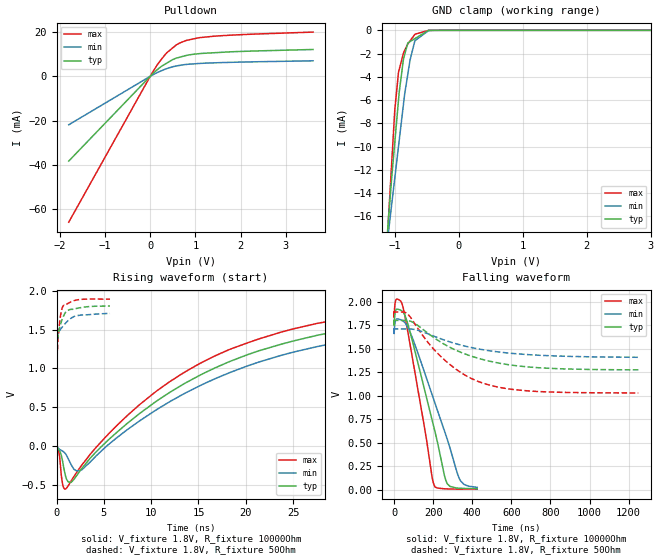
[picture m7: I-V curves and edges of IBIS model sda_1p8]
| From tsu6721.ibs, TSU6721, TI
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|   sda_1p8 Model
[Model]   sda_1p8
Model_type   I/O_open_drain
Polarity   Non-Inverting
Enable   Active-High
Vinl = 0.54
Vinh = 1.26
Vmeas = 0.9
Vref = 1.8
Cref = 35pF
Rref = 10000
|   typ   min   max
C_comp   1.376e-12   1.221e-12   1.514e-12
[Model spec]
|subparameter
Vinl   0.54   0.513   0.567
Vinh   1.26   1.197   1.323
[Voltage Range]   1.8   1.71   1.89
|Ambient Temperature   25   85   -40
|Junction Temperature
[Temperature Range]   27   125   -40
[Pullup Reference]   1.8   1.71   1.89
[Pulldown Reference]   0   0   0
[Power Clamp Reference]   1.8   1.71   1.89
[GND Clamp Reference]   0   0   0
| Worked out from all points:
|   slope of the pulldown table from 0 to 0.27 V, typ, clamps not added: 56.5 ohm
|   GND clamp passes 1 mA (typ) near -0.77 V on its own axis
|   falling waveform, V_fixture 1.8V, R_fixture 10000Ohm: 20-80 % time 125ns typ, 162ns min, 92.3ns max; typ from 1.8 V to 0.01 V
|   rising waveform, V_fixture 1.8V, R_fixture 10000Ohm: 20-80 % time 19.9ns typ, 21.8ns min, 17.8ns max; typ from 0.009 V to 1.8 V
|   falling waveform, V_fixture 1.8V, R_fixture 50Ohm: 20-80 % time 309ns typ, 337ns min, 257ns max; typ from 1.8 V to 1.27 V
|   rising waveform, V_fixture 1.8V, R_fixture 50Ohm: 20-80 % time 717ps typ, 1.33ns min, 398ps max; typ from 1.27 V to 1.8 V
[Pulldown]
|   Voltage   I(typ)   I(min)   I(max)
-1.8V     -38.2mA    -21.84mA   -65.75mA
35.91mV   716.9uA    418.8uA    1.294mA
168.2mV   3.206mA    1.819mA    5.583mA
332.6mV   5.544mA    3.231mA    9.865mA
574.6mV   8.199mA    4.667mA    14.12mA
797.6mV   9.416mA    5.363mA    16.19mA
1.058V    10.18mA    5.763mA    17.33mA
1.382V    10.6mA     6.059mA    18.03mA
3.6V      12.09mA    6.997mA    19.94mA
[GND Clamp]
|   Voltage   I(typ)   I(min)   I(max)
-1.8V     -71.23mA   -53.99mA   -101.6mA
-1.165V   -21.26mA   -20.52mA   -23.91mA
-1.096V   -16.21mA   -17.32mA   -16.16mA
-1.044V   -12.54mA   -14.88mA   -11.22mA
-999.8mV  -9.773mA   -12.81mA   -7.043mA
-939.3mV  -5.987mA   -9.974mA   -3.59mA
-862.2mV  -2.474mA   -6.361mA   -1.972mA
-793.8mV  -1.081mA   -3.757mA   -1.169mA
-759.2mV  -966.1uA   -2.551mA   -910.4uA
-682.3mV  -709.7uA   -893.4uA   -334.1uA
-434.3mV  -4.616uA   -12.32uA   -1.347uA
3.6V      0A         0A         0A
[POWER Clamp]
|   Voltage   I(typ)   I(min)   I(max)
-1.8V     0A         0A         0A
0V        0A         0A         0A
3.6V      0A         0A         0A
[Ramp]
R_load = 10000
|   typ   min   max
dV/dt_r   1.07486/1.99435e-08   1.01737/2.21728e-08   1.13092/1.78159e-08
dV/dt_f   1.07441/1.25188e-07   1.01502/1.6283e-07   1.13085/9.2297e-08
[Falling Waveform]
V_fixture = 1.8V
V_fixture_min = 1.71V
V_fixture_max = 1.89V
R_fixture = 10000Ohm
|   Time   V(typ)   V(min)   V(max)
0s        1.8V       1.71V      1.89V
200ps     1.747V     1.66V      1.832V
5.275ns   1.878V     1.777V     1.983V
13.03ns   1.92V      1.815V     2.027V
47.75ns   1.885V     1.792V     1.925V
96.45ns   1.561V     1.6V       1.371V
207.4ns   634.4mV    932mV      37.15mV
272.2ns   62.63mV    535.6mV    8.087mV
339.5ns   14.97mV    95.52mV    6.075mV
425.1ns   10.34mV    24.6mV     5.437mV
[Rising Waveform]
V_fixture = 1.8V
V_fixture_min = 1.71V
V_fixture_max = 1.89V
R_fixture = 10000Ohm
|   Time   V(typ)   V(min)   V(max)
0s        8.562mV    14.37mV    5.137mV
650ps     -195.2mV   -62.19mV   -491.8mV
925ps     -367.8mV   -92.12mV   -550mV
1.5ns     -464.7mV   -224.7mV   -453.8mV
2.625ns   -291.7mV   -303.7mV   -248.8mV
12ns      695.6mV    576mV      833.3mV
18.4ns    1.094V     951.8mV    1.25V
27.58ns   1.427V     1.282V     1.58V
45.83ns   1.705V     1.579V     1.83V
76.27ns   1.796V     1.698V     1.891V
[Falling Waveform]
V_fixture = 1.8V
V_fixture_min = 1.71V
V_fixture_max = 1.89V
R_fixture = 50Ohm
|   Time   V(typ)   V(min)   V(max)
0s        1.8V       1.71V      1.89V
69.63ns   1.798V     1.71V      1.868V
100.5ns   1.776V     1.705V     1.782V
173.7ns   1.663V     1.658V     1.566V
250.9ns   1.554V     1.596V     1.393V
351.4ns   1.453V     1.533V     1.233V
461ns     1.381V     1.486V     1.129V
587.4ns   1.329V     1.453V     1.072V
732.4ns   1.298V     1.431V     1.045V
1.25us    1.275V     1.408V     1.029V
[Rising Waveform]
V_fixture = 1.8V
V_fixture_min = 1.71V
V_fixture_max = 1.89V
R_fixture = 50Ohm
|   Time   V(typ)   V(min)   V(max)
0s        1.273V     1.406V     1.028V
25ps      1.266V     1.397V     1.032V
100ps     1.365V     1.431V     1.245V
150ps     1.414V     1.448V     1.349V
300ps     1.511V     1.483V     1.563V
500ps     1.596V     1.516V     1.73V
700ps     1.662V     1.546V     1.804V
1.125ns   1.742V     1.603V     1.829V
2.05ns    1.769V     1.676V     1.878V
5.65ns    1.801V     1.707V     1.891V
